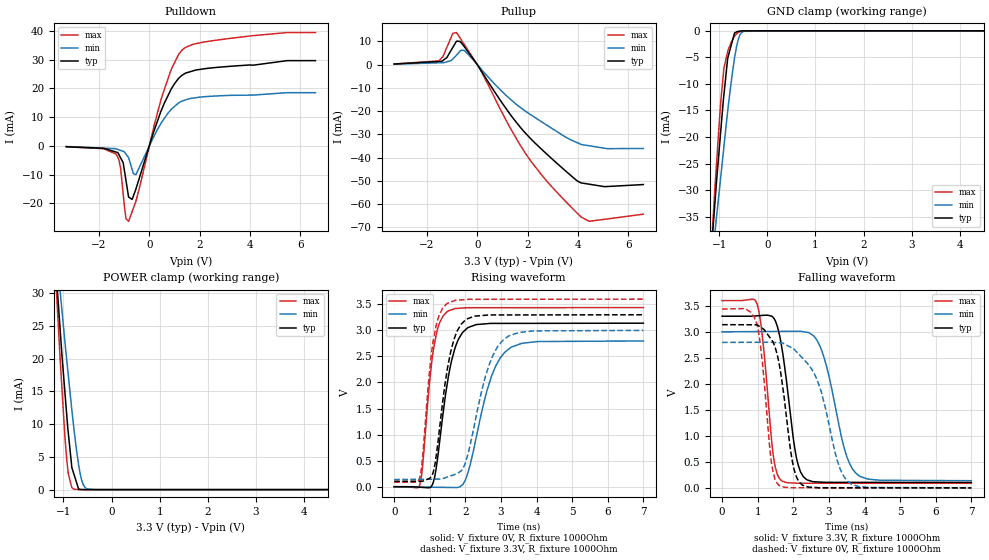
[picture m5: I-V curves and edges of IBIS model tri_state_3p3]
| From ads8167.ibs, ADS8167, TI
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|   tri_state_3p3 Model
[Model]   tri_state_3p3
Model_type   3-state
Polarity   Non-Inverting
Vmeas = 1.65
Vref = 0
Cref = 20pF
Rref = 250
|   typ   min   max
C_comp   1.2035E-12F   1.1675E-12F 1.2152E-12F
|  Where Nom  PVT is Nominal Process, 3.3V,   27C
|   Fast PVT is Strong Process,  3.6V,   -40C
|   Slow PVT is Weak Process,   3.0V,   125C
[Voltage Range]   3.3   3   3.6
|Junction Temperature
[Temperature Range]   27   125   -40
[Pullup Reference]   3.3   3   3.6
[Pulldown Reference]   -0   0   0
[Power Clamp Reference]   3.3   3   3.6
[GND Clamp Reference]   0   0   0
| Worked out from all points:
|   slope of the pulldown table from 0 to 0.495 V, typ, clamps not added: 38.9 ohm
|   slope of the pullup table from 0 to 0.495 V, typ, clamps not added: 58.4 ohm
|   GND clamp passes 1 mA (typ) near -0.70 V on its own axis
|   POWER clamp passes 1 mA (typ) near -0.72 V on its own axis
|   falling waveform, V_fixture 3.3V, R_fixture 1000Ohm: 20-80 % time 360ps typ, 558ps min, 276ps max; typ from 3.3 V to 0.103 V
|   rising waveform, V_fixture 0V, R_fixture 1000Ohm: 20-80 % time 413ps typ, 623ps min, 297ps max; typ from 0 V to 3.14 V
|   rising waveform, V_fixture 3.3V, R_fixture 1000Ohm: 20-80 % time 406ps typ, 616ps min, 296ps max; typ from 0.103 V to 3.3 V
|   falling waveform, V_fixture 0V, R_fixture 1000Ohm: 20-80 % time 379ps typ, 667ps min, 276ps max; typ from 3.14 V to 0 V
[Pulldown]
|   Voltage   I(typ)   I(min)   I(max)
-3.3V     -320.4uA   -242uA     -331.6uA
-1.322V   -2.174mA   -1.038mA   -2.84mA
-1.141V   -4.195mA   -1.601mA   -7.851mA
-1.039V   -5.901mA   -1.916mA   -16.78mA
-926.8mV  -12.14mA   -2.919mA   -25.41mA
-824.9mV  -17.81mA   -4.09mA    -26.26mA
-683.6mV  -18.64mA   -8.25mA    -22.9mA
-542mV    -15.27mA   -10.09mA   -19.53mA
513mV     13.1mA     8.497mA    17.48mA
1.296V    24.54mA    15.55mA    33.28mA
2.993V    27.5mA     17.47mA    37.13mA
6.6V      29.63mA    18.49mA    39.39mA
[GND Clamp]
|   Voltage   I(typ)   I(min)   I(max)
-3.3V     -311.7mA   -252.7mA   -388.5mA
-1.163V   -41.15mA   -44.21mA   -40.6mA
-1.085V   -31.82mA   -37.52mA   -28.86mA
-1.052V   -27.77mA   -34.62mA   -24.32mA
-973.2mV  -19.3mA    -27.85mA   -13.73mA
-903mV    -12.03mA   -21.8mA    -7.012mA
-824.9mV  -5.17mA    -15.08mA   -3.832mA
-683.6mV  -428.3uA   -5.193mA   -1.037mA
-635.7mV  -175.1uA   -2.785mA   -546.5uA
-540.6mV  -21.7uA    -371.3uA   -93.3uA
-322.3mV  -12.94uA   -829.7nA   -323.2nA
6.6V      0A         0A         0A
[Pullup]
|   Voltage   I(typ)   I(min)   I(max)
-3.3V     215.3uA    170.1uA    231.8uA
-1.524V   1.306mA    749.7uA    1.589mA
-1.211V   2.968mA    1.166mA    7.325mA
-970.6mV  7.373mA    2.419mA    13.42mA
-824.9mV  10.05mA    4.016mA    13.75mA
-520.3mV  7.768mA    6.07mA     8.71mA
115.5mV   -1.999mA   -1.46mA    -2.072mA
730.3mV   -12.37mA   -8.861mA   -15.19mA
1.964V    -30.06mA   -20.43mA   -38.96mA
4.125V    -50.89mA   -34.36mA   -65.55mA
4.451V    -51.46mA   -34.93mA   -67.4mA
6.6V      -51.6mA    -36.08mA   -64.34mA
[POWER Clamp]
|   Voltage   I(typ)   I(min)   I(max)
-3.3V     282mA      230.1mA    349.6mA
-1.135V   31.41mA    35.5mA     28.97mA
-1.074V   25.04mA    30.74mA    20.61mA
-1.03V    20.47mA    27.32mA    15.35mA
-932.5mV  11.49mA    19.91mA    4.653mA
-899.1mV  8.677mA    17.5mA     2.398mA
-824.9mV  3.359mA    12.13mA    324.9uA
-774.9mV  2.193mA    8.84mA     61.18uA
-683.6mV  65.69uA    3.756mA    6.412uA
-637.8mV  16.65uA    1.958mA    1.65uA
-503.9mV  349.2nA    87.36uA    718.3nA
6.6V      0A         0A         0A
[Ramp]
R_load = 1000
|   typ   min   max
dV/dt_r   1.88292/4.10556e-10   1.67827/6.18292e-10   2.06261/2.96187e-10
dV/dt_f   1.91814/3.58545e-10   1.71752/5.5411e-10   2.10699/2.75468e-10
[Falling Waveform]
V_fixture = 3.3V
V_fixture_min = 3V
V_fixture_max = 3.6V
R_fixture = 1000Ohm
C_fixture = 0F
|   Time   V(typ)   V(min)   V(max)
0s        3.3V       3V         3.6V
980.5ps   3.308V     3.005V     3.537V
1.149ns   3.317V     3.006V     2.802V
1.44ns    3.273V     3.008V     616.3mV
1.67ns    2.727V     3.009V     137.7mV
2.077ns   617.3mV    3.011V     90.56mV
2.367ns   161.7mV    2.993V     90.01mV
2.833ns   107.6mV    2.575V     89.85mV
3.751ns   105.5mV    286.8mV    89.51mV
7ns       103.1mV    137.4mV    88.34mV
[Rising Waveform]
V_fixture = 0V
V_fixture_min = 0V
V_fixture_max = 0V
R_fixture = 1000Ohm
C_fixture = 0F
|   Time   V(typ)   V(min)   V(max)
0s        6.039uV    123.4uV    -289.5nV
714.8ps   -9.754mV   -6.48mV    29.49mV
791.8ps   -13.02mV   -7.191mV   357mV
1.109ns   108.9mV    -10.12mV   2.656V
1.49ns    1.973V     -13.64mV   3.361V
1.697ns   2.637V     -15.56mV   3.417V
1.917ns   2.958V     37.03mV    3.429V
2.723ns   3.134V     2.099V     3.436V
3.281ns   3.134V     2.675V     3.436V
7ns       3.138V     2.797V     3.438V
[Rising Waveform]
V_fixture = 3.3V
V_fixture_min = 3V
V_fixture_max = 3.6V
R_fixture = 1000Ohm
C_fixture = 0F
|   Time   V(typ)   V(min)   V(max)
0s        103.1mV    137.5mV    88.34mV
714.8ps   104.8mV    142mV      168.7mV
1.099ns   286.1mV    144.4mV    2.807V
1.259ns   1.027V     145.4mV    3.281V
1.48ns    2.202V     182.5mV    3.512V
1.717ns   2.9V       238mV      3.576V
2.017ns   3.21V      499.5mV    3.592V
2.653ns   3.296V     2.312V     3.597V
3.191ns   3.296V     2.883V     3.597V
7ns       3.3V       3V         3.6V
[Falling Waveform]
|Gnd
V_fixture = 0V
V_fixture_min = 0V
V_fixture_max = 0V
R_fixture = 1000Ohm
C_fixture = 0F
|   Time   V(typ)   V(min)   V(max)
0s        3.138V     2.796V     3.438V
955.4ps   3.135V     2.799V     3.194V
1.119ns   3.073V     2.8V       2.494V
1.39ns    2.846V     2.799V     470.7mV
1.61ns    2.357V     2.789V     43.8mV
1.987ns   460.1mV    2.679V     2.774mV
2.257ns   53mV       2.495V     1.587mV
2.673ns   4.79mV     2.07V      1.448mV
3.621ns   2.282mV    76.44mV    1.131mV
7ns       6.066uV    122.9uV    -289.2nV
